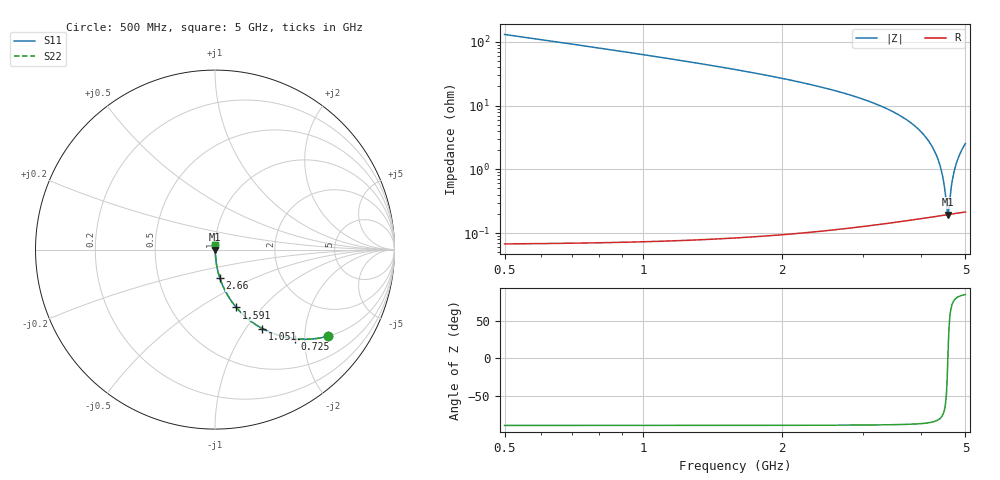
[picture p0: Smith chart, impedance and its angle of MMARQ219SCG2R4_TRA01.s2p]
! MMARQ219SCG2R4_TRA01  S-PARAMETER MODEL  ( General Type )
! Model Generated by TAIYO YUDEN Corporation (http://www.ty-top.com)
! Version 1.0
! TAIYO YUDEN Control No. 180601
! Copyright(c) 2018 TAIYO YUDEN CO.,LTD. All Rights Reserved.
! Product Description (link to TY-COMPAS)
! https://ds.yuden.co.jp/TYCOMPAS/or/detail?pn=MMARQ219SCG2R4BTRA01&u=M
! Products Name : Multilayer Ceramic Capacitors
! Characteristics :
!  Capacitance : 2.4 pF , Rated Voltage : 250V , TCC : CG / C0G
!  Case Size : 2.0 x 1.25 / 0.079 x 0.049 [mm/inch] , Thickness : 0.85 / 0.033 [mm/inch]
!  (Conditions: Temperature = 25 degC , DC Bias Current/Voltage = 0A / 0V)
! External Node Assignments :
!  1  o---| |---o  2
! GND o---------o GND
! Frequency Range : 500MHz  -  5000MHz  [ 401 STEP ]
# MHz S RI R 50
! Freq[MHz].  S11 Real  S11 Imag  S21 Real  S21 Imag  S12 Real  S12 Imag  S22 Real  S22 Imag
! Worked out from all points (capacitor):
!   401 points, 500 MHz to 5 GHz, reference 50 ohm
!   read as one part in series: C = 2.4 pF near 522.5 MHz
!   lowest |Z| = 195 mohm at 4.584 GHz (marker M1)
!   series resonance near 4.581 GHz, so ESL is about 500 pH
!   S11 on the Smith chart (normalised r, x): 500 MHz: 1.00, -2.62; 725 MHz: 1.00, -1.78; 1.051 GHz: 1.00, -1.20; 1.591 GHz: 1.00, -0.73; 2.66 GHz: 1.00, -0.33; 5 GHz: 1.00, +0.05
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500  0.632 -0.482  0.368 0.482  0.368 0.482  0.632 -0.482
725  0.443 -0.4964  0.557 0.4964  0.557 0.4964  0.443 -0.4964
1051.25  0.2634 -0.4398  0.7366 0.4398  0.7366 0.4398  0.2634 -0.4398
1253.75  0.1935 -0.3943  0.8065 0.3943  0.8065 0.3943  0.1935 -0.3943
1591.25  0.1189 -0.3225  0.8811 0.3225  0.8811 0.3225  0.1189 -0.3225
2007.5  0.0672 -0.2486  0.9328 0.2486  0.9328 0.2486  0.0672 -0.2486
2660  0.0276 -0.1603  0.9724 0.1603  0.9724 0.1603  0.0276 -0.1603
2750  0.0243 -0.1501  0.9757 0.1501  0.9757 0.1501  0.0243 -0.1501
3503.75  0.00754 -0.0777  0.9925 0.0777  0.9925 0.0777  0.00754 -0.0777
3953.75  0.00346 -0.0425  0.9965 0.0425  0.9965 0.0425  0.00346 -0.0425
4122.5  0.00265 -0.0304  0.9973 0.0304  0.9973 0.0304  0.00265 -0.0304
4257.5  0.00223 -0.0211  0.9978 0.0211  0.9978 0.0211  0.00223 -0.0211
4358.75  0.00204 -0.0143  0.998 0.0143  0.998 0.0143  0.00204 -0.0143
4437.5  0.00196 -0.00915  0.998 0.00915  0.998 0.00915  0.00196 -0.00915
4493.75  0.00193 -0.00553  0.9981 0.00553  0.9981 0.00553  0.00193 -0.00553
4561.25  0.00193 -0.00124  0.9981 0.00124  0.9981 0.00124  0.00193 -0.00124
4583.75  0.00194 0.000174  0.9981 -0.000174  0.9981 -0.000174  0.00194 0.000174
4606.25  0.00195 0.00158  0.998 -0.00158  0.998 -0.00158  0.00195 0.00158
4673.75  0.00201 0.00576  0.998 -0.00576  0.998 -0.00576  0.00201 0.00576
4741.25  0.00211 0.00988  0.9979 -0.00988  0.9979 -0.00988  0.00211 0.00988
4853.75  0.00234 0.0166  0.9977 -0.0166  0.9977 -0.0166  0.00234 0.0166
5000  0.00277 0.0252  0.9972 -0.0252  0.9972 -0.0252  0.00277 0.0252
